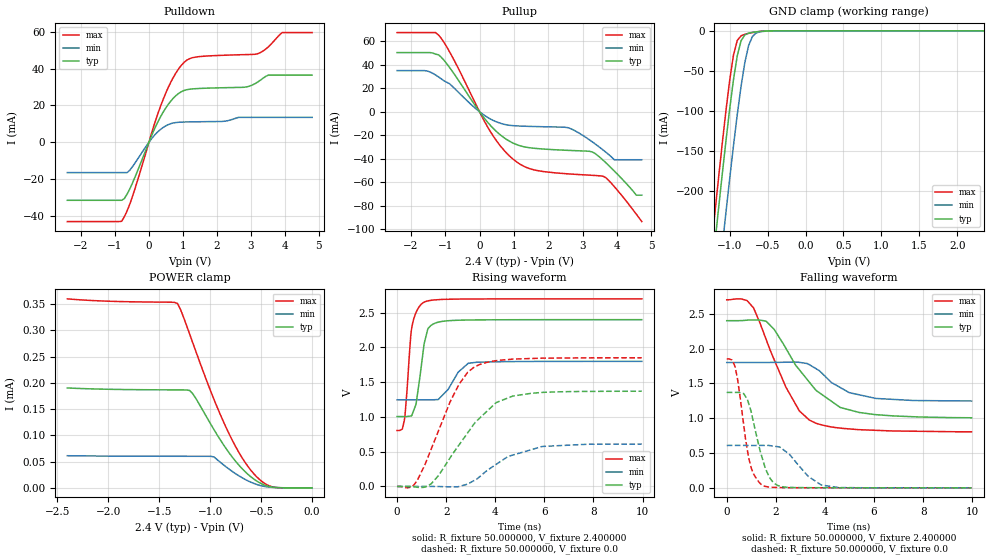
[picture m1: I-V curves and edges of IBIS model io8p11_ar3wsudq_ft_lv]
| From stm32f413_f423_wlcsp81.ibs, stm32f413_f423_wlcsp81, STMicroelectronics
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|   Model io8p11_ar3wsudq_ft_lv
[Model]  io8p11_ar3wsudq_ft_lv
Model_type I/O
Polarity   Non-Inverting
Enable   Active-Low
Vinl =   0.720000V
Vinh =   1.680000V
Vmeas =  1.200000V
Cref =   30.000000pF
Rref =   100.000000M
Vref =   0.0V
C_comp   3.740800pF   3.684200pF   3.822900pF
[Temperature Range]   25.000000   0.125000k   -40.000000
[Pullup Reference]   2.400000V   1.800000V   2.700000V
[Pulldown Reference]   0.0V   0.0V   0.0V
[POWER Clamp Reference]   2.400000V   1.800000V   2.700000V
[GND Clamp Reference]   0.0V   0.0V   0.0V
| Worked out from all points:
|   slope of the pulldown table from 0 to 0.36 V, typ, clamps not added: 25 ohm
|   slope of the pullup table from 0 to 0.36 V, typ, clamps not added: 27.7 ohm
|   GND clamp passes 1 mA (typ) near -0.62 V on its own axis
|   rising waveform, R_fixture 50.000000, V_fixture 2.400000: 20-80 % time 337ps typ, 660ps min, 257ps max; typ from 1.01 V to 2.4 V
|   rising waveform, R_fixture 50.000000, V_fixture 0.0: 20-80 % time 1.8ns typ, 1.76ns min, 1.35ns max; typ from 0 V to 1.37 V
|   falling waveform, R_fixture 50.000000, V_fixture 2.400000: 20-80 % time 1.89ns typ, 1.37ns min, 1.43ns max; typ from 2.4 V to 1.01 V
|   falling waveform, R_fixture 50.000000, V_fixture 0.0: 20-80 % time 588ps typ, 968ps min, 464ps max; typ from 1.37 V to 0 V
[Pulldown]
|Voltage   I(typ)   I(min)   I(max)
-2.4V     -31.47mA   -16.45mA   -43.01mA
-800mV    -31.47mA   -16.45mA   -42.85mA
-480mV    -21.98mA   -13.17mA   -29.21mA
80mV      3.63mA     1.966mA    5.014mA
480mV     18.16mA    8.738mA    26.02mA
800mV     25.38mA    10.72mA    37.77mA
1.12V     28.53mA    11.02mA    44.6mA
2.8V      29.84mA    13.51mA    47.53mA
3.2V      32.66mA    13.51mA    48.04mA
3.52V     36.44mA    13.51mA    51.84mA
3.92V     36.44mA    13.51mA    59.5mA
4.8V      36.44mA    13.51mA    59.5mA
[Pullup]
|Voltage   I(typ)   I(min)   I(max)
-2.4V     50.45mA    35.09mA    67.51mA
-1.52V    50.45mA    34.74mA    67.51mA
-1.2V     48.65mA    29.87mA    65.66mA
320mV     -11.75mA   -6.207mA   -17.08mA
1.04V     -27.54mA   -11.97mA   -41.91mA
1.6V      -31.14mA   -12.58mA   -49.63mA
2.56V     -32.88mA   -13.52mA   -52.9mA
3.28V     -34.25mA   -25.64mA   -54.18mA
3.6V      -41.44mA   -32.74mA   -55.03mA
3.92V     -50.46mA   -40.9mA    -63.79mA
4.56V     -71.1mA    -40.9mA    -87.27mA
4.72V     -71.1mA    -40.9mA    -93.6mA
[GND_clamp]
|Voltage   I(typ)   I(min)   I(max)
-2.4V     -1.429A    -1.514A    -1.399A
-1.25V    -315.9mA   -407.2mA   -278.2mA
-1.2V     -270.1mA   -361.3mA   -232.1mA
-1.15V    -225mA     -316mA     -186.8mA
-1.1V     -180.9mA   -271.3mA   -142.7mA
-1.05V    -138.2mA   -227.5mA   -100.5mA
-950mV    -61.14mA   -143.6mA   -30.43mA
-900mV    -31.23mA   -104.7mA   -12.14mA
-850mV    -12.49mA   -69.4mA    -6.221mA
-750mV    -2.898mA   -18.35mA   -3.18mA
-600mV    -750.2uA   -1.218mA   -738.3uA
2.35V     0A         0A         0A
[POWER_clamp]
|Voltage   I(typ)   I(min)   I(max)
-2.4V     190.2uA    61.19uA    359.9uA
-1.32V    186.6uA    60.14uA    351.2uA
-1.29V    186.5uA    60.13uA    339.6uA
-1.2V     185.4uA    60.11uA    292.6uA
-1.17V    179.2uA    60.11uA    276.3uA
-960mV    110.2uA    58.62uA    167.5uA
-870mV    82.44uA    43.99uA    126.3uA
-750mV    50.58uA    26.92uA    78.64uA
-630mV    25.94uA    13.41uA    41.02uA
-510mV    9.22uA     4.527uA    14.97uA
-420mV    2.425uA    1.38uA     3.75uA
0V        0A         0A         0A
[Ramp]
| variable   typ   min   max
dV/dt_r  0.82176/1.79371n   0.36392/1.74958n   1.11108/1.34673n
dV/dt_f  0.83316/1.88622n   0.33246/1.39533n   1.13576/1.42763n
R_load = 50.000000
[Rising Waveform]
R_fixture= 50.000000
V_fixture= 2.400000
V_fixture_min= 1.800000
V_fixture_max= 2.700000
|time   V(typ)   V(min)   V(max)
0s        1.006V     1.247V     804.7mV
220.2ps   1.006V     1.247V     829.8mV
320.3ps   1.006V     1.247V     1.001V
600.6ps   1.02V      1.247V     2.283V
780.8ps   1.198V     1.247V     2.507V
1.081ns   1.988V     1.247V     2.648V
1.261ns   2.273V     1.246V     2.67V
1.461ns   2.335V     1.247V     2.682V
2.903ns   2.395V     1.772V     2.697V
9.97ns    2.4V       1.8V       2.699V
[Rising Waveform]
R_fixture= 50.000000
V_fixture= 0.0
V_fixture_min= 0.0
V_fixture_max= 0.0
|time   V(typ)   V(min)   V(max)
0s        164.7uV    65.06uV    284.1uV
540.5ps   -1.32mV    51.37uV    -12.07mV
820.8ps   -11.83mV   61.75uV    83.34mV
1.401ns   40.83mV    135.7uV    546.1mV
2.182ns   422.2mV    -6.889mV   1.231V
3.143ns   902.2mV    85.61mV    1.716V
4.044ns   1.208V     319mV      1.81V
4.725ns   1.301V     452.2mV    1.832V
5.926ns   1.353V     575.4mV    1.846V
9.97ns    1.37V      609mV      1.851V
[Falling Waveform]
R_fixture= 50.000000
V_fixture= 2.400000
V_fixture_min= 1.800000
V_fixture_max= 2.700000
|time   V(typ)   V(min)   V(max)
0s        2.4V       1.8V       2.699V
820.8ps   2.407V     1.8V       2.689V
1.101ns   2.41V      1.8V       2.577V
1.602ns   2.393V     1.8V       2.134V
2.402ns   2.008V     1.804V     1.451V
2.963ns   1.693V     1.801V     1.103V
3.363ns   1.518V     1.768V     973.9mV
4.625ns   1.154V     1.44V      857.6mV
5.385ns   1.083V     1.337V     835.2mV
9.97ns    1.006V     1.247V     804.7mV
[Falling Waveform]
R_fixture= 50.000000
V_fixture= 0.0
V_fixture_min= 0.0
V_fixture_max= 0.0
|time   V(typ)   V(min)   V(max)
0s        1.37V      609mV      1.851V
340.3ps   1.37V      609mV      1.735V
440.4ps   1.37V      609mV      1.561V
840.8ps   1.268V     608.9mV    543mV
1.081ns   955.9mV    608.7mV    210.5mV
1.441ns   434.5mV    609.1mV    39.75mV
1.722ns   162.4mV    608.1mV    11.7mV
2.042ns   40.98mV    592.4mV    5.379mV
3.864ns   1.758mV    39.73mV    1.119mV
9.97ns    164.7uV    65.06uV    284.1uV
